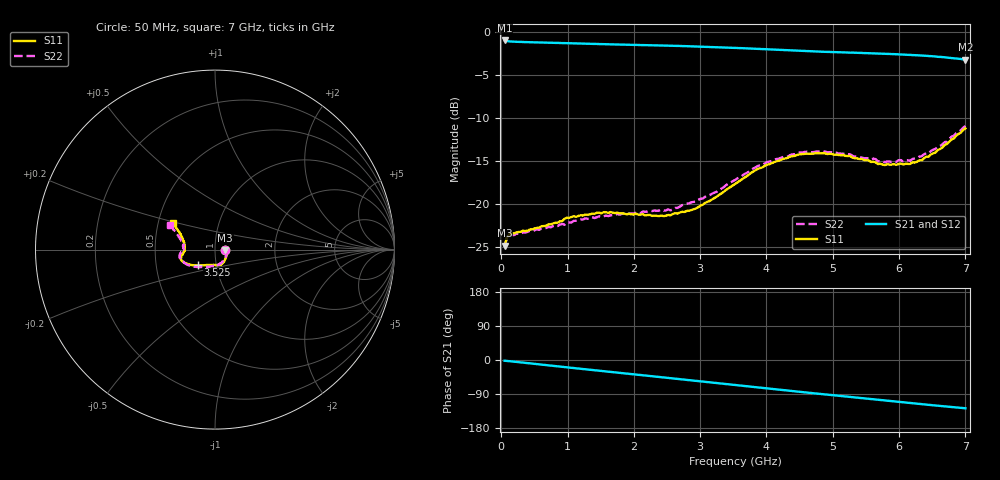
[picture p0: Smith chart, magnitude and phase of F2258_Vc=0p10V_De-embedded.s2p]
! Integrated Device Technology
! Corporate Headquarters
! 6024 Silver Creek Valley Road
! San Jose, CA 95138  USA
! Phone:  1-408-284-8200
! Toll Free:  1-800-223-1366
! Webpage:  http://www.idt.com/
! Timing and RF Division
! 515 Groton Road, Suite 102
! Westford, MA 01886-6024
! Device:  F2258
! Description: Voltage Variable RF Attenuator
! Frequency:  50.0 -  6000.00 MHz
! Package:  3x3 mm Thin QFN Plastic Package: 16 pin
! Ports:  2 RF, 2 DC
!  Pin  1  = NC
!  Pin  2  = NC
!  Pin  3  = RF2  = Port 2
!  Pin  4  = GND
!  Pin  5  = Vdd
!  Pin  6  = NC
!  Pin  7  = VCTRL
!  Pin  8  = NC
!  Pin  9  = GND
!  Pin 10  = RF1  = Port 1
!  Pin 11  = NC
!  Pin 12  = NC
!  Pin 13  = NC
!  Pin 14  = NC
!  Pin 15  = NC
!  Pin 16  = NC
! Vcntrl:  0.100 Volts
! Vdd:  +3.300 Volts
! Current:  1.076 mA
! Data:  The device was measured on a the F2258 evaluation board which has
!  individual transmission lines to the RF pins.  Data was collected
!  using a calibrated network analyzer.  The evaluation board was
!  de-embedded using a TRL calibration technique.
!  The reference plane is the edge of the package pin.
! Misc:  SN 10
!  Action Tracker AT0285
! Date Measured:  2014-12-10
! Date:  2016-01-13  MJV
! Note:
!  Integrated Device Technology supplies this data as a sample of measured
!  data at the package pin for this product.  Your particular data for this
!  product may vary.
!  Data was taken at 25 degrees C.
!  Integrated Device Technology reserves the right to change this data at anytime.
!Freq_(GHz)  S11M_(dB)  S11P_(deg)  S21M_(dB)  S21P_(deg)  S12M_(dB)  S12P_(deg)  S22M_(dB)  S22P_(deg)
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# GHz S dB R 50
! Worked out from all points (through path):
!   201 points, 50 MHz to 7 GHz, reference 50 ohm
!   highest |S21| = -0.96 dB at 50 MHz (marker M1); lowest = -3.2 dB at 7 GHz (marker M2)
!   group delay of S21, straight-line fit = 50.5 ps
!   lowest |S11| = -24.9 dB at 50 MHz (marker M3), VSWR 1.12, Z = 56 - j0.388 ohm
!   |S11| at or under -10 dB: start of sweep to end of sweep
!   |S22| runs from -24.9 to -10.9 dB; largest |S21 - S12| = 0.00044
!   S11 on the Smith chart (normalised r, x): 50 MHz: 1.12, -0.01; 3.525 GHz: 0.81, -0.14; 7 GHz: 0.60, +0.19
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0.05  -24.88 -3.5  -0.96 -1.9  -0.96 -1.9  -24.91 -3.1
0.08475  -23.90 -6.0  -1.03 -2.4  -1.03 -2.4  -23.99 -5.5
0.15425  -23.41 -9.2  -1.08 -3.6  -1.08 -3.6  -23.60 -9.4
0.71025  -22.39 -37.2  -1.22 -14.1  -1.22 -14.1  -22.69 -38.6
0.91875  -21.99 -47.0  -1.26 -18.0  -1.26 -18.0  -22.33 -50.4
0.98825  -21.60 -51.0  -1.27 -19.3  -1.27 -19.3  -22.17 -54.7
1.2315  -21.35 -59.3  -1.32 -23.8  -1.32 -23.8  -21.80 -63.7
1.6485  -20.94 -71.0  -1.41 -31.4  -1.41 -31.4  -21.31 -76.7
2.37825  -21.42 -92.4  -1.54 -44.8  -1.54 -44.7  -20.78 -94.3
2.552  -21.31 -98.4  -1.57 -48.0  -1.57 -48.0  -20.74 -99.6
2.93425  -20.53 -115.1  -1.65 -55.1  -1.65 -55.1  -19.73 -112.9
3.525  -17.69 -137.8  -1.82 -66.2  -1.82 -66.2  -17.21 -135.6
4.0115  -15.43 -151.3  -2.00 -75.2  -2.00 -75.2  -15.12 -151.0
4.46325  -14.28 -159.8  -2.16 -83.4  -2.16 -83.4  -14.07 -162.1
4.7065  -14.14 -163.1  -2.23 -87.7  -2.23 -87.7  -13.96 -166.3
5.2625  -14.43 -170.0  -2.38 -97.4  -2.38 -97.3  -14.21 -174.3
5.6795  -15.35 -176.8  -2.47 -104.6  -2.47 -104.6  -15.03 -179.6
5.85325  -15.41 179.0  -2.52 -107.8  -2.52 -107.8  -15.06 175.7
6.166  -15.34 171.2  -2.63 -113.4  -2.63 -113.3  -14.97 169.8
6.33975  -14.93 164.9  -2.71 -116.5  -2.71 -116.5  -14.43 165.4
6.722  -13.01 153.3  -2.94 -123.1  -2.94 -123.1  -12.71 156.4
7  -11.20 147.9  -3.19 -127.4  -3.19 -127.4  -10.92 151.5
